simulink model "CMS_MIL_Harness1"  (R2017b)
settings: Solver=FixedStepDiscrete  StartTime=0.0  StopTime=23  FixedStep=0.01  RelTol=1e-3  EnableMultiTasking=on
undefined symbols (not defined in the file): sigbuilder_block
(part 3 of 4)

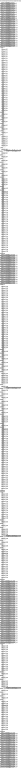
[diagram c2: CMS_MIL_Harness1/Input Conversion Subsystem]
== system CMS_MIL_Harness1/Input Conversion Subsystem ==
  note: This subsystem has been inserted by Simulink to adapt the output of the source blocks to the interface required by the harnessed component. Modifying the contents of this subsystem may result in compilation and simulation failure.
  Inport_1 : Inport
  Inport_2 : Inport  Port=2
  Inport_3 : Inport  Port=3
  Inport_4 : Inport  Port=4
  Inport_5 : Inport  Port=5
  Inport_6 : Inport  Port=6
  Inport_7 : Inport  Port=7
  Inport_8 : Inport  Port=8
  Inport_9 : Inport  Port=9
  Inport_10 : Inport  Port=10
  Inport_11 : Inport  Port=11
  Inport_12 : Inport  Port=12
  Inport_13 : Inport  Port=13
  Inport_14 : Inport  Port=14
  Inport_15 : Inport  Port=15
  Inport_16 : Inport  Port=16
  Inport_17 : Inport  Port=17
  Inport_18 : Inport  Port=18
  Inport_19 : Inport  Port=19
  Inport_20 : Inport  Port=20
  Inport_21 : Inport  Port=21
  Inport_22 : Inport  Port=22
  Inport_23 : Inport  Port=23
  Inport_24 : Inport  Port=24
  Inport_25 : Inport  Port=25
  Inport_26 : Inport  Port=26
  Inport_27 : Inport  Port=27
  Inport_28 : Inport  Port=28
  Inport_29 : Inport  Port=29
  Inport_30 : Inport  Port=30
  Inport_31 : Inport  Port=31
  Inport_32 : Inport  Port=32
  Inport_33 : Inport  Port=33
  Inport_34 : Inport  Port=34
  Inport_35 : Inport  Port=35
  Inport_36 : Inport  Port=36
  Inport_37 : Inport  Port=37
  Inport_38 : Inport  Port=38
  Inport_39 : Inport  Port=39
  Inport_40 : Inport  Port=40
  Inport_41 : Inport  Port=41
  Inport_42 : Inport  Port=42
  Inport_43 : Inport  Port=43
  Inport_44 : Inport  Port=44
  Inport_45 : Inport  Port=45
  Inport_46 : Inport  Port=46
  Inport_47 : Inport  Port=47
  Inport_48 : Inport  Port=48
  Inport_49 : Inport  Port=49
  Inport_50 : Inport  Port=50
  Inport_51 : Inport  Port=51
  Inport_52 : Inport  Port=52
  Inport_53 : Inport  Port=53
  Inport_54 : Inport  Port=54
  Inport_55 : Inport  Port=55
  Inport_56 : Inport  Port=56
  Inport_57 : Inport  Port=57
  Inport_58 : Inport  Port=58
  Inport_59 : Inport  Port=59
  Inport_60 : Inport  Port=60
  Inport_61 : Inport  Port=61
  Inport_62 : Inport  Port=62
  Inport_63 : Inport  Port=63
  Inport_64 : Inport  Port=64
  Inport_65 : Inport  Port=65
  Inport_66 : Inport  Port=66
  Inport_67 : Inport  Port=67
  Inport_68 : Inport  Port=68
  Inport_69 : Inport  Port=69
  Inport_70 : Inport  Port=70
  Inport_71 : Inport  Port=71
  Inport_72 : Inport  Port=72
  Inport_73 : Inport  Port=73
  Inport_74 : Inport  Port=74
  Inport_75 : Inport  Port=75
  Inport_76 : Inport  Port=76
  Inport_77 : Inport  Port=77
  Inport_78 : Inport  Port=78
  Inport_79 : Inport  Port=79
  Inport_80 : Inport  Port=80
  Inport_81 : Inport  Port=81
  Inport_82 : Inport  Port=82
  Inport_83 : Inport  Port=83
  Inport_84 : Inport  Port=84
  Inport_85 : Inport  Port=85
  Inport_86 : Inport  Port=86
  Inport_87 : Inport  Port=87
  Inport_88 : Inport  Port=88
  Inport_89 : Inport  Port=89
  Inport_90 : Inport  Port=90
  Inport_91 : Inport  Port=91
  Inport_92 : Inport  Port=92
  Inport_93 : Inport  Port=93
  Inport_94 : Inport  Port=94
  Inport_95 : Inport  Port=95
  Inport_96 : Inport  Port=96
  Inport_97 : Inport  Port=97
  Inport_98 : Inport  Port=98
  Inport_99 : Inport  Port=99
  Inport_100 : Inport  Port=100
  Inport_101 : Inport  Port=101
  Inport_102 : Inport  Port=102
  Inport_103 : Inport  Port=103
  Inport_104 : Inport  Port=104
  Inport_105 : Inport  Port=105
  Inport_106 : Inport  Port=106
  Inport_107 : Inport  Port=107
  Inport_108 : Inport  Port=108
  Inport_109 : Inport  Port=109
  Inport_110 : Inport  Port=110
  Inport_111 : Inport  Port=111
  Inport_112 : Inport  Port=112
  Inport_113 : Inport  Port=113
  Inport_114 : Inport  Port=114
  Inport_115 : Inport  Port=115
  Inport_116 : Inport  Port=116
  Inport_117 : Inport  Port=117
  Inport_118 : Inport  Port=118
  Inport_119 : Inport  Port=119
  Inport_120 : Inport  Port=120
  Inport_121 : Inport  Port=121
  Inport_122 : Inport  Port=122
  Inport_123 : Inport  Port=123
  Inport_124 : Inport  Port=124
  Inport_125 : Inport  Port=125
  Inport_126 : Inport  Port=126
  Inport_127 : Inport  Port=127
  Inport_128 : Inport  Port=128
  Inport_129 : Inport  Port=129
  Inport_130 : Inport  Port=130
  Inport_131 : Inport  Port=131
  Inport_132 : Inport  Port=132
  Inport_133 : Inport  Port=133
  Inport_134 : Inport  Port=134
  Inport_135 : Inport  Port=135
  Inport_136 : Inport  Port=136
  Inport_137 : Inport  Port=137
  Inport_138 : Inport  Port=138
  Inport_139 : Inport  Port=139
  Inport_140 : Inport  Port=140
  Inport_141 : Inport  Port=141
  Inport_142 : Inport  Port=142
  Inport_143 : Inport  Port=143
  Inport_144 : Inport  Port=144
  Inport_145 : Inport  Port=145
  Inport_146 : Inport  Port=146
  Inport_147 : Inport  Port=147
  Inport_148 : Inport  Port=148
  Inport_149 : Inport  Port=149
  Inport_150 : Inport  Port=150
  Inport_151 : Inport  Port=151
  Inport_152 : Inport  Port=152
  Inport_153 : Inport  Port=153
  Inport_154 : Inport  Port=154
  Inport_155 : Inport  Port=155
  Inport_156 : Inport  Port=156
  Inport_157 : Inport  Port=157
  Inport_158 : Inport  Port=158
  Inport_159 : Inport  Port=159
  Inport_160 : Inport  Port=160
  Inport_161 : Inport  Port=161
  Inport_162 : Inport  Port=162
  Inport_163 : Inport  Port=163
  Inport_164 : Inport  Port=164
  Inport_165 : Inport  Port=165
  Inport_166 : Inport  Port=166
  Inport_167 : Inport  Port=167
  Inport_168 : Inport  Port=168
  Inport_169 : Inport  Port=169
  Inport_170 : Inport  Port=170
  Inport_171 : Inport  Port=171
  Inport_172 : Inport  Port=172
  Inport_173 : Inport  Port=173
  Inport_174 : Inport  Port=174
  Inport_175 : Inport  Port=175
  Inport_176 : Inport  Port=176
  Inport_177 : Inport  Port=177
  Inport_178 : Inport  Port=178
  Inport_179 : Inport  Port=179
  Inport_180 : Inport  Port=180
  Inport_181 : Inport  Port=181
  Inport_182 : Inport  Port=182
  Inport_183 : Inport  Port=183
  Inport_184 : Inport  Port=184
  Inport_185 : Inport  Port=185
  Inport_186 : Inport  Port=186
  Inport_187 : Inport  Port=187
  Inport_188 : Inport  Port=188
  Inport_189 : Inport  Port=189
  Inport_190 : Inport  Port=190
  Inport_191 : Inport  Port=191
  Inport_192 : Inport  Port=192
  Inport_193 : Inport  Port=193
  Inport_194 : Inport  Port=194
  Inport_195 : Inport  Port=195
  Inport_196 : Inport  Port=196
  Inport_197 : Inport  Port=197
  Inport_198 : Inport  Port=198
  Inport_199 : Inport  Port=199
  Inport_200 : Inport  Port=200
  Inport_201 : Inport  Port=201
  Inport_202 : Inport  Port=202
  Inport_203 : Inport  Port=203
  Inport_204 : Inport  Port=204
  Inport_205 : Inport  Port=205
  Inport_206 : Inport  Port=206
  Inport_207 : Inport  Port=207
  Inport_208 : Inport  Port=208
  Inport_209 : Inport  Port=209
  Inport_210 : Inport  Port=210
  Inport_211 : Inport  Port=211
  Inport_212 : Inport  Port=212
  Inport_213 : Inport  Port=213
  Inport_214 : Inport  Port=214
  Inport_215 : Inport  Port=215
  Inport_216 : Inport  Port=216
  Inport_217 : Inport  Port=217
  Inport_218 : Inport  Port=218
  Inport_219 : Inport  Port=219
  Inport_220 : Inport  Port=220
  Inport_221 : Inport  Port=221
  Inport_222 : Inport  Port=222
  Inport_223 : Inport  Port=223
  Inport_224 : Inport  Port=224
  Inport_225 : Inport  Port=225
  Inport_226 : Inport  Port=226
  Inport_227 : Inport  Port=227
  Inport_228 : Inport  Port=228
  Inport_229 : Inport  Port=229
  Inport_230 : Inport  Port=230
  Inport_231 : Inport  Port=231
  Inport_232 : Inport  Port=232
  Inport_233 : Inport  Port=233
  Inport_234 : Inport  Port=234
  Inport_235 : Inport  Port=235
  Inport_236 : Inport  Port=236
  Inport_237 : Inport  Port=237
  Inport_238 : Inport  Port=238
  Inport_239 : Inport  Port=239
  Inport_240 : Inport  Port=240
  Inport_241 : Inport  Port=241
  Inport_242 : Inport  Port=242
  Inport_243 : Inport  Port=243
  Inport_244 : Inport  Port=244
  Inport_245 : Inport  Port=245
  Inport_246 : Inport  Port=246
  Inport_247 : Inport  Port=247
  Inport_248 : Inport  Port=248
  Inport_249 : Inport  Port=249
  Inport_250 : Inport  Port=250
  Inport_251 : Inport  Port=251
  Inport_252 : Inport  Port=252
  Inport_253 : Inport  Port=253
  Inport_254 : Inport  Port=254
  Inport_255 : Inport  Port=255
  Inport_256 : Inport  Port=256
  Inport_257 : Inport  Port=257
  Inport_258 : Inport  Port=258
  Inport_259 : Inport  Port=259
  Inport_260 : Inport  Port=260
  Inport_261 : Inport  Port=261
  Inport_262 : Inport  Port=262
  Inport_263 : Inport  Port=263
  Inport_264 : Inport  Port=264
  Inport_265 : Inport  Port=265
  Inport_266 : Inport  Port=266
  Inport_267 : Inport  Port=267
  Inport_268 : Inport  Port=268
  Inport_269 : Inport  Port=269
  Inport_270 : Inport  Port=270
  Inport_271 : Inport  Port=271
  Inport_272 : Inport  Port=272
  Inport_273 : Inport  Port=273
  Inport_274 : Inport  Port=274
  Inport_275 : Inport  Port=275
  Inport_276 : Inport  Port=276
  Inport_277 : Inport  Port=277
  Inport_278 : Inport  Port=278
  Inport_279 : Inport  Port=279
  Inport_280 : Inport  Port=280
  Inport_281 : Inport  Port=281
  Inport_282 : Inport  Port=282
  Inport_283 : Inport  Port=283
  Inport_284 : Inport  Port=284
  Inport_285 : Inport  Port=285
  Inport_286 : Inport  Port=286
  Inport_287 : Inport  Port=287
  Inport_288 : Inport  Port=288
  Inport_289 : Inport  Port=289
  Inport_290 : Inport  Port=290
  Inport_291 : Inport  Port=291
  Inport_292 : Inport  Port=292
  Inport_293 : Inport  Port=293
  Inport_294 : Inport  Port=294
  Inport_295 : Inport  Port=295
  Inport_296 : Inport  Port=296
  Inport_297 : Inport  Port=297
  Inport_298 : Inport  Port=298
  Inport_299 : Inport  Port=299
  Inport_300 : Inport  Port=300
  Inport_301 : Inport  Port=301
  Inport_302 : Inport  Port=302
  Inport_303 : Inport  Port=303
  Inport_304 : Inport  Port=304
  Inport_305 : Inport  Port=305
  Inport_306 : Inport  Port=306
  Inport_307 : Inport  Port=307
  Inport_308 : Inport  Port=308
  Inport_309 : Inport  Port=309
  Inport_310 : Inport  Port=310
  Inport_311 : Inport  Port=311
  Inport_312 : Inport  Port=312
  Inport_313 : Inport  Port=313
  Inport_314 : Inport  Port=314
  Inport_315 : Inport  Port=315
  Inport_316 : Inport  Port=316
  Inport_317 : Inport  Port=317
  Inport_318 : Inport  Port=318
  Inport_319 : Inport  Port=319
  Inport_320 : Inport  Port=320
  Inport_321 : Inport  Port=321
  Inport_322 : Inport  Port=322
  Inport_323 : Inport  Port=323
  Inport_324 : Inport  Port=324
  Inport_325 : Inport  Port=325
  Inport_326 : Inport  Port=326
  Inport_327 : Inport  Port=327
  Inport_328 : Inport  Port=328
  Inport_329 : Inport  Port=329
  Inport_330 : Inport  Port=330
  Inport_331 : Inport  Port=331
  Inport_332 : Inport  Port=332
  Inport_333 : Inport  Port=333
  Inport_334 : Inport  Port=334
  Inport_335 : Inport  Port=335
  Inport_336 : Inport  Port=336
  Inport_337 : Inport  Port=337
  Inport_338 : Inport  Port=338
  Inport_339 : Inport  Port=339
  Inport_340 : Inport  Port=340
  Inport_341 : Inport  Port=341
  Inport_342 : Inport  Port=342
  Inport_343 : Inport  Port=343
  Inport_344 : Inport  Port=344
  Inport_345 : Inport  Port=345
  Inport_346 : Inport  Port=346
  Inport_347 : Inport  Port=347
  Inport_348 : Inport  Port=348
  Inport_349 : Inport  Port=349
  Inport_350 : Inport  Port=350
  Inport_351 : Inport  Port=351
  Inport_352 : Inport  Port=352
  Inport_353 : Inport  Port=353
  Inport_354 : Inport  Port=354
  Inport_355 : Inport  Port=355
  Inport_356 : Inport  Port=356
  Inport_357 : Inport  Port=357
  Inport_358 : Inport  Port=358
  Inport_359 : Inport  Port=359
  Inport_360 : Inport  Port=360
  Inport_361 : Inport  Port=361
  Inport_362 : Inport  Port=362
  Inport_363 : Inport  Port=363
  Inport_364 : Inport  Port=364
  Inport_365 : Inport  Port=365
  Inport_366 : Inport  Port=366
  Inport_367 : Inport  Port=367
  Inport_368 : Inport  Port=368
  Inport_369 : Inport  Port=369
  Inport_370 : Inport  Port=370
  Inport_371 : Inport  Port=371
  Inport_372 : Inport  Port=372
  Inport_373 : Inport  Port=373
  Inport_374 : Inport  Port=374
  Inport_375 : Inport  Port=375
  Inport_376 : Inport  Port=376
  Inport_377 : Inport  Port=377
  Inport_378 : Inport  Port=378
  Inport_379 : Inport  Port=379
  Inport_380 : Inport  Port=380
  Inport_381 : Inport  Port=381
  Inport_382 : Inport  Port=382
  Inport_383 : Inport  Port=383
  Inport_384 : Inport  Port=384
  Inport_385 : Inport  Port=385
  Inport_386 : Inport  Port=386
  Inport_387 : Inport  Port=387
  Inport_388 : Inport  Port=388
  Inport_389 : Inport  Port=389
  Inport_390 : Inport  Port=390
  Inport_391 : Inport  Port=391
  Inport_392 : Inport  Port=392
  Inport_393 : Inport  Port=393
  Inport_394 : Inport  Port=394
  Inport_395 : Inport  Port=395
  Inport_396 : Inport  Port=396
  Inport_397 : Inport  Port=397
  Inport_398 : Inport  Port=398
  Inport_399 : Inport  Port=399
  Inport_400 : Inport  Port=400
  Inport_401 : Inport  Port=401
  Inport_402 : Inport  Port=402
  Inport_403 : Inport  Port=403
  Inport_404 : Inport  Port=404
  Inport_405 : Inport  Port=405
  Inport_406 : Inport  Port=406
  Inport_407 : Inport  Port=407
  Inport_408 : Inport  Port=408
  Inport_409 : Inport  Port=409
  Inport_410 : Inport  Port=410
  Inport_411 : Inport  Port=411
  Inport_412 : Inport  Port=412
  Inport_413 : Inport  Port=413
  Concat_1 : Concatenate  NumInputs=112
  Concat_2 : Concatenate  NumInputs=112
  Concat_3 : Concatenate  NumInputs=48
  Concat_4 : Concatenate  NumInputs=48
  Data_Conversion_{1,16,20,31,34..36,51..52,54,58..61,73,78..79,83..85,99..101} (23 alike) : DataTypeConversion  OutDataTypeStr=uint8
  Data_Conversion_{10..11,30,43,71..72,86} (7 alike) : DataTypeConversion  OutDataTypeStr=uint16
  Data_Conversion_{2..5,7,9,12,15,17,19,24..25,27,32..33,38,53,56,62..64,67..68,80,87..88,91..98} (34 alike) : DataTypeConversion  OutDataTypeStr=boolean
  Data_Conversion_{6,8,13..14,18,21..23,28..29,37,39..40,42,45,47..50,55,57,65..66,69..70,74..77,81,89..90} (32 alike) : DataTypeConversion  OutDataTypeStr=single
  Data_Conversion_26 : Reshape  OutputDimensionality=Customize  OutputDimensions=[112]
  Data_Conversion_41 : DataTypeConversion  OutDataTypeStr=fixdt('ufix16_Sp1')
  Data_Conversion_44 : Reshape  OutputDimensionality=Customize  OutputDimensions=[112]
  Data_Conversion_46 : Reshape  OutputDimensionality=Customize  OutputDimensions=[48]
  Data_Conversion_82 : Reshape  OutputDimensionality=Customize  OutputDimensions=[48]
  RateTs_{1..97} (97 alike) : RateTransition  OutPortSampleTime=0.01
  SigSpec_{1,16,20,33..35,48..49,51,70,75,95..97} (14 alike) : SignalSpecification  OutDataTypeStr=uint8  Unit=enum  Dimensions=[1]  SampleTime=0.01
  SigSpec_10 : SignalSpecification  OutDataTypeStr=uint16  Unit=mV  Dimensions=[1]  SampleTime=0.01
  SigSpec_11 : SignalSpecification  OutDataTypeStr=uint16  Unit=mV  Dimensions=[1]  SampleTime=0.01
  SigSpec_{12,15,17,19,24,26,31..32,37,50,60..61,64..65,77,83..84,87..93} (24 alike) : SignalSpecification  OutDataTypeStr=boolean  Unit=flag  Dimensions=[1]  SampleTime=0.01
  SigSpec_{6,13,52,54,63,85} (6 alike) : SignalSpecification  OutDataTypeStr=single  Unit=V  Dimensions=[1]  SampleTime=0.01
  SigSpec_{8,14,23,41,62,86} (6 alike) : SignalSpecification  OutDataTypeStr=single  Unit=A  Dimensions=[1]  SampleTime=0.01
  SigSpec_18 : SignalSpecification  OutDataTypeStr=single  Unit=pct  Dimensions=[1]  SampleTime=0.01
  SigSpec_{2..5,7,9,53,59,94} (9 alike) : SignalSpecification  OutDataTypeStr=boolean  Unit=flg  Dimensions=[1]  SampleTime=0.01
  SigSpec_21 : SignalSpecification  OutDataTypeStr=single  Unit=pct  Dimensions=[1]  SampleTime=0.01
  SigSpec_22 : SignalSpecification  OutDataTypeStr=single  Unit=pct  Dimensions=[1]  SampleTime=0.01
  SigSpec_25 : SignalSpecification  OutDataTypeStr=boolean  Unit=flag  Dimensions=[112]  SampleTime=0.01
  SigSpec_{27..28,71..72} (4 alike) : SignalSpecification  OutDataTypeStr=single  Unit=kW  Dimensions=[1]  SampleTime=0.01
  SigSpec_29 : SignalSpecification  OutDataTypeStr=uint16  Unit=kohm  Dimensions=[1]  SampleTime=0.01
  SigSpec_{30,55..58,76,79..81} (9 alike) : SignalSpecification  OutDataTypeStr=uint8  Unit=numb  Dimensions=[1]  SampleTime=0.01
  SigSpec_{36,38..39,44..45,66..67,73..74} (9 alike) : SignalSpecification  OutDataTypeStr=single  Unit=C  Dimensions=[1]  SampleTime=0.01
  SigSpec_40 : SignalSpecification  OutDataTypeStr=fixdt('ufix16_Sp1')  Unit=V  Dimensions=[1]  SampleTime=0.01
  SigSpec_42 : SignalSpecification  OutDataTypeStr=uint16  Unit=mV  Dimensions=[112]  SampleTime=0.01
  SigSpec_43 : SignalSpecification  OutDataTypeStr=single  Unit=C  Dimensions=[48]  SampleTime=0.01
  SigSpec_46 : SignalSpecification  OutDataTypeStr=single  Unit=W  Dimensions=[1]  SampleTime=0.01
  SigSpec_47 : SignalSpecification  OutDataTypeStr=single  Unit=W  Dimensions=[1]  SampleTime=0.01
  SigSpec_68 : SignalSpecification  OutDataTypeStr=uint16  Unit=min  Dimensions=[1]  SampleTime=0.01
  SigSpec_69 : SignalSpecification  OutDataTypeStr=uint16  Unit=min  Dimensions=[1]  SampleTime=0.01
  SigSpec_78 : SignalSpecification  OutDataTypeStr=single  Unit=C  Dimensions=[48]  SampleTime=0.01
  SigSpec_82 : SignalSpecification  OutDataTypeStr=uint16  Unit=kWh  Dimensions=[1]  SampleTime=0.01
  Outport_1 : Outport
  Outport_2 : Outport  Port=2
  Outport_3 : Outport  Port=3
  Outport_4 : Outport  Port=4
  Outport_5 : Outport  Port=5
  Outport_6 : Outport  Port=6
  Outport_7 : Outport  Port=7
  Outport_8 : Outport  Port=8
  Outport_9 : Outport  Port=9
  Outport_10 : Outport  Port=10
  Outport_11 : Outport  Port=11
  Outport_12 : Outport  Port=12
  Outport_13 : Outport  Port=13
  Outport_14 : Outport  Port=14
  Outport_15 : Outport  Port=15
  Outport_16 : Outport  Port=16
  Outport_17 : Outport  Port=17
  Outport_18 : Outport  Port=18
  Outport_19 : Outport  Port=19
  Outport_20 : Outport  Port=20
  Outport_21 : Outport  Port=21
  Outport_22 : Outport  Port=22
  Outport_23 : Outport  Port=23
  Outport_24 : Outport  Port=24
  Outport_25 : Outport  Port=25
  Outport_26 : Outport  Port=26
  Outport_27 : Outport  Port=27
  Outport_28 : Outport  Port=28
  Outport_29 : Outport  Port=29
  Outport_30 : Outport  Port=30
  Outport_31 : Outport  Port=31
  Outport_32 : Outport  Port=32
  Outport_33 : Outport  Port=33
  Outport_34 : Outport  Port=34
  Outport_35 : Outport  Port=35
  Outport_36 : Outport  Port=36
  Outport_37 : Outport  Port=37
  Outport_38 : Outport  Port=38
  Outport_39 : Outport  Port=39
  Outport_40 : Outport  Port=40
  Outport_41 : Outport  Port=41
  Outport_42 : Outport  Port=42
  Outport_43 : Outport  Port=43
  Outport_44 : Outport  Port=44
  Outport_45 : Outport  Port=45
  Outport_46 : Outport  Port=46
  Outport_47 : Outport  Port=47
  Outport_48 : Outport  Port=48
  Outport_49 : Outport  Port=49
  Outport_50 : Outport  Port=50
  Outport_51 : Outport  Port=51
  Outport_52 : Outport  Port=52
  Outport_53 : Outport  Port=53
  Outport_54 : Outport  Port=54
  Outport_55 : Outport  Port=55
  Outport_56 : Outport  Port=56
  Outport_57 : Outport  Port=57
  Outport_58 : Outport  Port=58
  Outport_59 : Outport  Port=59
  Outport_60 : Outport  Port=60
  Outport_61 : Outport  Port=61
  Outport_62 : Outport  Port=62
  Outport_63 : Outport  Port=63
  Outport_64 : Outport  Port=64
  Outport_65 : Outport  Port=65
  Outport_66 : Outport  Port=66
  Outport_67 : Outport  Port=67
  Outport_68 : Outport  Port=68
  Outport_69 : Outport  Port=69
  Outport_70 : Outport  Port=70
  Outport_71 : Outport  Port=71
  Outport_72 : Outport  Port=72
  Outport_73 : Outport  Port=73
  Outport_74 : Outport  Port=74
  Outport_75 : Outport  Port=75
  Outport_76 : Outport  Port=76
  Outport_77 : Outport  Port=77
  Outport_78 : Outport  Port=78
  Outport_79 : Outport  Port=79
  Outport_80 : Outport  Port=80
  Outport_81 : Outport  Port=81
  Outport_82 : Outport  Port=82
  Outport_83 : Outport  Port=83
  Outport_84 : Outport  Port=84
  Outport_85 : Outport  Port=85
  Outport_86 : Outport  Port=86
  Outport_87 : Outport  Port=87
  Outport_88 : Outport  Port=88
  Outport_89 : Outport  Port=89
  Outport_90 : Outport  Port=90
  Outport_91 : Outport  Port=91
  Outport_92 : Outport  Port=92
  Outport_93 : Outport  Port=93
  Outport_94 : Outport  Port=94
  Outport_95 : Outport  Port=95
  Outport_96 : Outport  Port=96
  Outport_97 : Outport  Port=97
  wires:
  SigSpec_1/1 -> Outport_1/1
  RateTs_1/1 -> SigSpec_1/1
  Data_Conversion_1/1 -> RateTs_1/1
  Inport_1/1 -> Data_Conversion_1/1
  SigSpec_2/1 -> Outport_2/1
  RateTs_2/1 -> SigSpec_2/1
  Data_Conversion_2/1 -> RateTs_2/1
  Inport_2/1 -> Data_Conversion_2/1
  SigSpec_3/1 -> Outport_3/1
  RateTs_3/1 -> SigSpec_3/1
  Data_Conversion_3/1 -> RateTs_3/1
  Inport_3/1 -> Data_Conversion_3/1
  SigSpec_4/1 -> Outport_4/1
  RateTs_4/1 -> SigSpec_4/1
  Data_Conversion_4/1 -> RateTs_4/1
  Inport_4/1 -> Data_Conversion_4/1
  SigSpec_5/1 -> Outport_5/1
  RateTs_5/1 -> SigSpec_5/1
  Data_Conversion_5/1 -> RateTs_5/1
  Inport_5/1 -> Data_Conversion_5/1
  SigSpec_6/1 -> Outport_6/1
  RateTs_6/1 -> SigSpec_6/1
  Data_Conversion_6/1 -> RateTs_6/1
  Inport_6/1 -> Data_Conversion_6/1
  SigSpec_7/1 -> Outport_7/1
  RateTs_7/1 -> SigSpec_7/1
  Data_Conversion_7/1 -> RateTs_7/1
  Inport_7/1 -> Data_Conversion_7/1
  SigSpec_8/1 -> Outport_8/1
  RateTs_8/1 -> SigSpec_8/1
  Data_Conversion_8/1 -> RateTs_8/1
  Inport_8/1 -> Data_Conversion_8/1
  SigSpec_9/1 -> Outport_9/1
  RateTs_9/1 -> SigSpec_9/1
  Data_Conversion_9/1 -> RateTs_9/1
  Inport_9/1 -> Data_Conversion_9/1
  SigSpec_10/1 -> Outport_10/1
  RateTs_10/1 -> SigSpec_10/1
  Data_Conversion_10/1 -> RateTs_10/1
  Inport_10/1 -> Data_Conversion_10/1
  SigSpec_11/1 -> Outport_11/1
  RateTs_11/1 -> SigSpec_11/1
  Data_Conversion_11/1 -> RateTs_11/1
  Inport_11/1 -> Data_Conversion_11/1
  SigSpec_12/1 -> Outport_12/1
  RateTs_12/1 -> SigSpec_12/1
  Data_Conversion_12/1 -> RateTs_12/1
  Inport_12/1 -> Data_Conversion_12/1
  SigSpec_13/1 -> Outport_13/1
  RateTs_13/1 -> SigSpec_13/1
  Data_Conversion_13/1 -> RateTs_13/1
  Inport_13/1 -> Data_Conversion_13/1
  SigSpec_14/1 -> Outport_14/1
  RateTs_14/1 -> SigSpec_14/1
  Data_Conversion_14/1 -> RateTs_14/1
  Inport_14/1 -> Data_Conversion_14/1
  SigSpec_15/1 -> Outport_15/1
  RateTs_15/1 -> SigSpec_15/1
  Data_Conversion_15/1 -> RateTs_15/1
  Inport_15/1 -> Data_Conversion_15/1
  SigSpec_16/1 -> Outport_16/1
  RateTs_16/1 -> SigSpec_16/1
  Data_Conversion_16/1 -> RateTs_16/1
  Inport_16/1 -> Data_Conversion_16/1
  SigSpec_17/1 -> Outport_17/1
  RateTs_17/1 -> SigSpec_17/1
  Data_Conversion_17/1 -> RateTs_17/1
  Inport_17/1 -> Data_Conversion_17/1
  SigSpec_18/1 -> Outport_18/1
  RateTs_18/1 -> SigSpec_18/1
  Data_Conversion_18/1 -> RateTs_18/1
  Inport_18/1 -> Data_Conversion_18/1
  SigSpec_19/1 -> Outport_19/1
  RateTs_19/1 -> SigSpec_19/1
  Data_Conversion_19/1 -> RateTs_19/1
  Inport_19/1 -> Data_Conversion_19/1
  SigSpec_20/1 -> Outport_20/1
  RateTs_20/1 -> SigSpec_20/1
  Data_Conversion_20/1 -> RateTs_20/1
  Inport_20/1 -> Data_Conversion_20/1
  SigSpec_21/1 -> Outport_21/1
  RateTs_21/1 -> SigSpec_21/1
  Data_Conversion_21/1 -> RateTs_21/1
  Inport_21/1 -> Data_Conversion_21/1
  SigSpec_22/1 -> Outport_22/1
  RateTs_22/1 -> SigSpec_22/1
  Data_Conversion_22/1 -> RateTs_22/1
  Inport_22/1 -> Data_Conversion_22/1
  SigSpec_23/1 -> Outport_23/1
  RateTs_23/1 -> SigSpec_23/1
  Data_Conversion_23/1 -> RateTs_23/1
  Inport_23/1 -> Data_Conversion_23/1
  SigSpec_24/1 -> Outport_24/1
  RateTs_24/1 -> SigSpec_24/1
  Data_Conversion_24/1 -> RateTs_24/1
  Inport_24/1 -> Data_Conversion_24/1
  SigSpec_25/1 -> Outport_25/1
  RateTs_25/1 -> SigSpec_25/1
  Data_Conversion_25/1 -> RateTs_25/1
  Data_Conversion_26/1 -> Data_Conversion_25/1
  Concat_1/1 -> Data_Conversion_26/1
  Inport_25/1 -> Concat_1/1
  Inport_26/1 -> Concat_1/2
  Inport_27/1 -> Concat_1/3
  Inport_28/1 -> Concat_1/4
  Inport_29/1 -> Concat_1/5
  Inport_30/1 -> Concat_1/6
  Inport_31/1 -> Concat_1/7
  Inport_32/1 -> Concat_1/8
  Inport_33/1 -> Concat_1/9
  Inport_34/1 -> Concat_1/10
  Inport_35/1 -> Concat_1/11
  Inport_36/1 -> Concat_1/12
  Inport_37/1 -> Concat_1/13
  Inport_38/1 -> Concat_1/14
  Inport_39/1 -> Concat_1/15
  Inport_40/1 -> Concat_1/16
  Inport_41/1 -> Concat_1/17
  Inport_42/1 -> Concat_1/18
  Inport_43/1 -> Concat_1/19
  Inport_44/1 -> Concat_1/20
  Inport_45/1 -> Concat_1/21
  Inport_46/1 -> Concat_1/22
  Inport_47/1 -> Concat_1/23
  Inport_48/1 -> Concat_1/24
  Inport_49/1 -> Concat_1/25
  Inport_50/1 -> Concat_1/26
  Inport_51/1 -> Concat_1/27
  Inport_52/1 -> Concat_1/28
  Inport_53/1 -> Concat_1/29
  Inport_54/1 -> Concat_1/30
  Inport_55/1 -> Concat_1/31
  Inport_56/1 -> Concat_1/32
  Inport_57/1 -> Concat_1/33
  Inport_58/1 -> Concat_1/34
  Inport_59/1 -> Concat_1/35
  Inport_60/1 -> Concat_1/36
  Inport_61/1 -> Concat_1/37
  Inport_62/1 -> Concat_1/38
  Inport_63/1 -> Concat_1/39
  Inport_64/1 -> Concat_1/40
  Inport_65/1 -> Concat_1/41
  Inport_66/1 -> Concat_1/42
  Inport_67/1 -> Concat_1/43
  Inport_68/1 -> Concat_1/44
  Inport_69/1 -> Concat_1/45
  Inport_70/1 -> Concat_1/46
  Inport_71/1 -> Concat_1/47
  Inport_72/1 -> Concat_1/48
  Inport_73/1 -> Concat_1/49
  Inport_74/1 -> Concat_1/50
  Inport_75/1 -> Concat_1/51
  Inport_76/1 -> Concat_1/52
  Inport_77/1 -> Concat_1/53
  Inport_78/1 -> Concat_1/54
  Inport_79/1 -> Concat_1/55
  Inport_80/1 -> Concat_1/56
  Inport_81/1 -> Concat_1/57
  Inport_82/1 -> Concat_1/58
  Inport_83/1 -> Concat_1/59
  Inport_84/1 -> Concat_1/60
  Inport_85/1 -> Concat_1/61
  Inport_86/1 -> Concat_1/62
  Inport_87/1 -> Concat_1/63
  Inport_88/1 -> Concat_1/64
  Inport_89/1 -> Concat_1/65
  Inport_90/1 -> Concat_1/66
  Inport_91/1 -> Concat_1/67
  Inport_92/1 -> Concat_1/68
  Inport_93/1 -> Concat_1/69
  Inport_94/1 -> Concat_1/70
  Inport_95/1 -> Concat_1/71
  Inport_96/1 -> Concat_1/72
  Inport_97/1 -> Concat_1/73
  Inport_98/1 -> Concat_1/74
  Inport_99/1 -> Concat_1/75
  Inport_100/1 -> Concat_1/76
  Inport_101/1 -> Concat_1/77
  Inport_102/1 -> Concat_1/78
  Inport_103/1 -> Concat_1/79
  Inport_104/1 -> Concat_1/80
  Inport_105/1 -> Concat_1/81
  Inport_106/1 -> Concat_1/82
  Inport_107/1 -> Concat_1/83
  Inport_108/1 -> Concat_1/84
  Inport_109/1 -> Concat_1/85
  Inport_110/1 -> Concat_1/86
  Inport_111/1 -> Concat_1/87
  Inport_112/1 -> Concat_1/88
  Inport_113/1 -> Concat_1/89
  Inport_114/1 -> Concat_1/90
  Inport_115/1 -> Concat_1/91
  Inport_116/1 -> Concat_1/92
  Inport_117/1 -> Concat_1/93
  Inport_118/1 -> Concat_1/94
  Inport_119/1 -> Concat_1/95
  Inport_120/1 -> Concat_1/96
  Inport_121/1 -> Concat_1/97
  Inport_122/1 -> Concat_1/98
  Inport_123/1 -> Concat_1/99
  Inport_124/1 -> Concat_1/100
  Inport_125/1 -> Concat_1/101
  Inport_126/1 -> Concat_1/102
  Inport_127/1 -> Concat_1/103
  Inport_128/1 -> Concat_1/104
  Inport_129/1 -> Concat_1/105
  Inport_130/1 -> Concat_1/106
  Inport_131/1 -> Concat_1/107
  Inport_132/1 -> Concat_1/108
  Inport_133/1 -> Concat_1/109
  Inport_134/1 -> Concat_1/110
  Inport_135/1 -> Concat_1/111
  Inport_136/1 -> Concat_1/112
  SigSpec_26/1 -> Outport_26/1
  RateTs_26/1 -> SigSpec_26/1
  Data_Conversion_27/1 -> RateTs_26/1
  Inport_137/1 -> Data_Conversion_27/1
  SigSpec_27/1 -> Outport_27/1
  RateTs_27/1 -> SigSpec_27/1
  Data_Conversion_28/1 -> RateTs_27/1
  Inport_138/1 -> Data_Conversion_28/1
  SigSpec_28/1 -> Outport_28/1
  RateTs_28/1 -> SigSpec_28/1
  Data_Conversion_29/1 -> RateTs_28/1
  Inport_139/1 -> Data_Conversion_29/1
  SigSpec_29/1 -> Outport_29/1
  RateTs_29/1 -> SigSpec_29/1
  Data_Conversion_30/1 -> RateTs_29/1
  Inport_140/1 -> Data_Conversion_30/1
  SigSpec_30/1 -> Outport_30/1
  RateTs_30/1 -> SigSpec_30/1
  Data_Conversion_31/1 -> RateTs_30/1
  Inport_141/1 -> Data_Conversion_31/1
  SigSpec_31/1 -> Outport_31/1
  RateTs_31/1 -> SigSpec_31/1
  Data_Conversion_32/1 -> RateTs_31/1
  Inport_142/1 -> Data_Conversion_32/1
  SigSpec_32/1 -> Outport_32/1
  RateTs_32/1 -> SigSpec_32/1
  Data_Conversion_33/1 -> RateTs_32/1
  Inport_143/1 -> Data_Conversion_33/1
  SigSpec_33/1 -> Outport_33/1
  RateTs_33/1 -> SigSpec_33/1
  Data_Conversion_34/1 -> RateTs_33/1
  Inport_144/1 -> Data_Conversion_34/1
  SigSpec_34/1 -> Outport_34/1
  RateTs_34/1 -> SigSpec_34/1
  Data_Conversion_35/1 -> RateTs_34/1
  Inport_145/1 -> Data_Conversion_35/1
  SigSpec_35/1 -> Outport_35/1
  RateTs_35/1 -> SigSpec_35/1
  Data_Conversion_36/1 -> RateTs_35/1
  Inport_146/1 -> Data_Conversion_36/1
  SigSpec_36/1 -> Outport_36/1
  RateTs_36/1 -> SigSpec_36/1
  Data_Conversion_37/1 -> RateTs_36/1
  Inport_147/1 -> Data_Conversion_37/1
  SigSpec_37/1 -> Outport_37/1
  RateTs_37/1 -> SigSpec_37/1
  Data_Conversion_38/1 -> RateTs_37/1
  Inport_148/1 -> Data_Conversion_38/1
  SigSpec_38/1 -> Outport_38/1
  RateTs_38/1 -> SigSpec_38/1
  Data_Conversion_39/1 -> RateTs_38/1
  Inport_149/1 -> Data_Conversion_39/1
  SigSpec_39/1 -> Outport_39/1
  RateTs_39/1 -> SigSpec_39/1
  Data_Conversion_40/1 -> RateTs_39/1
  Inport_150/1 -> Data_Conversion_40/1
  SigSpec_40/1 -> Outport_40/1
  RateTs_40/1 -> SigSpec_40/1
  Data_Conversion_41/1 -> RateTs_40/1
  Inport_151/1 -> Data_Conversion_41/1
  SigSpec_41/1 -> Outport_41/1
  RateTs_41/1 -> SigSpec_41/1
  Data_Conversion_42/1 -> RateTs_41/1
  Inport_152/1 -> Data_Conversion_42/1
  SigSpec_42/1 -> Outport_42/1
  RateTs_42/1 -> SigSpec_42/1
  Data_Conversion_43/1 -> RateTs_42/1
  Data_Conversion_44/1 -> Data_Conversion_43/1
  Concat_2/1 -> Data_Conversion_44/1
  Inport_153/1 -> Concat_2/1
  Inport_154/1 -> Concat_2/2
  Inport_155/1 -> Concat_2/3
  Inport_156/1 -> Concat_2/4
  Inport_157/1 -> Concat_2/5
  Inport_158/1 -> Concat_2/6
  Inport_159/1 -> Concat_2/7
  Inport_160/1 -> Concat_2/8
  Inport_161/1 -> Concat_2/9
  Inport_162/1 -> Concat_2/10
  Inport_163/1 -> Concat_2/11
  Inport_164/1 -> Concat_2/12
  Inport_165/1 -> Concat_2/13
  Inport_166/1 -> Concat_2/14
  Inport_167/1 -> Concat_2/15
  Inport_168/1 -> Concat_2/16
  Inport_169/1 -> Concat_2/17
  Inport_170/1 -> Concat_2/18
  Inport_171/1 -> Concat_2/19
  Inport_172/1 -> Concat_2/20
  Inport_173/1 -> Concat_2/21
  Inport_174/1 -> Concat_2/22
  Inport_175/1 -> Concat_2/23
  Inport_176/1 -> Concat_2/24
  Inport_177/1 -> Concat_2/25
  Inport_178/1 -> Concat_2/26
  Inport_179/1 -> Concat_2/27
  Inport_180/1 -> Concat_2/28
  Inport_181/1 -> Concat_2/29
  Inport_182/1 -> Concat_2/30
  Inport_183/1 -> Concat_2/31
  Inport_184/1 -> Concat_2/32
  Inport_185/1 -> Concat_2/33
  Inport_186/1 -> Concat_2/34
  Inport_187/1 -> Concat_2/35
  Inport_188/1 -> Concat_2/36
  Inport_189/1 -> Concat_2/37
  Inport_190/1 -> Concat_2/38
  Inport_191/1 -> Concat_2/39
  Inport_192/1 -> Concat_2/40
  Inport_193/1 -> Concat_2/41
  Inport_194/1 -> Concat_2/42
  Inport_195/1 -> Concat_2/43
  Inport_196/1 -> Concat_2/44
  Inport_197/1 -> Concat_2/45
  Inport_198/1 -> Concat_2/46
  Inport_199/1 -> Concat_2/47
  Inport_200/1 -> Concat_2/48
  Inport_201/1 -> Concat_2/49
  Inport_202/1 -> Concat_2/50
  Inport_203/1 -> Concat_2/51
  Inport_204/1 -> Concat_2/52
  Inport_205/1 -> Concat_2/53
  Inport_206/1 -> Concat_2/54
  Inport_207/1 -> Concat_2/55
  Inport_208/1 -> Concat_2/56
  Inport_209/1 -> Concat_2/57
  Inport_210/1 -> Concat_2/58
  Inport_211/1 -> Concat_2/59
  Inport_212/1 -> Concat_2/60
  Inport_213/1 -> Concat_2/61
  Inport_214/1 -> Concat_2/62
  Inport_215/1 -> Concat_2/63
  Inport_216/1 -> Concat_2/64
  Inport_217/1 -> Concat_2/65
  Inport_218/1 -> Concat_2/66
  Inport_219/1 -> Concat_2/67
  Inport_220/1 -> Concat_2/68
  Inport_221/1 -> Concat_2/69
  Inport_222/1 -> Concat_2/70
  Inport_223/1 -> Concat_2/71
  Inport_224/1 -> Concat_2/72
  Inport_225/1 -> Concat_2/73
  Inport_226/1 -> Concat_2/74
  Inport_227/1 -> Concat_2/75
  Inport_228/1 -> Concat_2/76
  Inport_229/1 -> Concat_2/77
  Inport_230/1 -> Concat_2/78
  Inport_231/1 -> Concat_2/79
  Inport_232/1 -> Concat_2/80
  Inport_233/1 -> Concat_2/81
  Inport_234/1 -> Concat_2/82
  Inport_235/1 -> Concat_2/83
  Inport_236/1 -> Concat_2/84
  Inport_237/1 -> Concat_2/85
  Inport_238/1 -> Concat_2/86
  Inport_239/1 -> Concat_2/87
  Inport_240/1 -> Concat_2/88
  Inport_241/1 -> Concat_2/89
  Inport_242/1 -> Concat_2/90
  Inport_243/1 -> Concat_2/91
  Inport_244/1 -> Concat_2/92
  Inport_245/1 -> Concat_2/93
  Inport_246/1 -> Concat_2/94
  Inport_247/1 -> Concat_2/95
  Inport_248/1 -> Concat_2/96
  Inport_249/1 -> Concat_2/97
  Inport_250/1 -> Concat_2/98
  Inport_251/1 -> Concat_2/99
  Inport_252/1 -> Concat_2/100
  Inport_253/1 -> Concat_2/101
  Inport_254/1 -> Concat_2/102
  Inport_255/1 -> Concat_2/103
  Inport_256/1 -> Concat_2/104
  Inport_257/1 -> Concat_2/105
  Inport_258/1 -> Concat_2/106
  Inport_259/1 -> Concat_2/107
  Inport_260/1 -> Concat_2/108
  Inport_261/1 -> Concat_2/109
  Inport_262/1 -> Concat_2/110
  Inport_263/1 -> Concat_2/111
  Inport_264/1 -> Concat_2/112
  SigSpec_43/1 -> Outport_43/1
  RateTs_43/1 -> SigSpec_43/1
  Data_Conversion_45/1 -> RateTs_43/1
  Data_Conversion_46/1 -> Data_Conversion_45/1
  Concat_3/1 -> Data_Conversion_46/1
  Inport_265/1 -> Concat_3/1
  Inport_266/1 -> Concat_3/2
  Inport_267/1 -> Concat_3/3
  Inport_268/1 -> Concat_3/4
  Inport_269/1 -> Concat_3/5
  Inport_270/1 -> Concat_3/6
  Inport_271/1 -> Concat_3/7
  Inport_272/1 -> Concat_3/8
  Inport_273/1 -> Concat_3/9
  Inport_274/1 -> Concat_3/10
  Inport_275/1 -> Concat_3/11
  Inport_276/1 -> Concat_3/12
  Inport_277/1 -> Concat_3/13
  Inport_278/1 -> Concat_3/14
  Inport_279/1 -> Concat_3/15
  Inport_280/1 -> Concat_3/16
  Inport_281/1 -> Concat_3/17
  Inport_282/1 -> Concat_3/18
  Inport_283/1 -> Concat_3/19
  Inport_284/1 -> Concat_3/20
  Inport_285/1 -> Concat_3/21
  Inport_286/1 -> Concat_3/22
  Inport_287/1 -> Concat_3/23
  Inport_288/1 -> Concat_3/24
  Inport_289/1 -> Concat_3/25
  Inport_290/1 -> Concat_3/26
  Inport_291/1 -> Concat_3/27
  Inport_292/1 -> Concat_3/28
  Inport_293/1 -> Concat_3/29
  Inport_294/1 -> Concat_3/30
  Inport_295/1 -> Concat_3/31
  Inport_296/1 -> Concat_3/32
  Inport_297/1 -> Concat_3/33
  Inport_298/1 -> Concat_3/34
  Inport_299/1 -> Concat_3/35
  Inport_300/1 -> Concat_3/36
  Inport_301/1 -> Concat_3/37
  Inport_302/1 -> Concat_3/38
  Inport_303/1 -> Concat_3/39
  Inport_304/1 -> Concat_3/40
  Inport_305/1 -> Concat_3/41
  Inport_306/1 -> Concat_3/42
  Inport_307/1 -> Concat_3/43
  Inport_308/1 -> Concat_3/44
  Inport_309/1 -> Concat_3/45
  Inport_310/1 -> Concat_3/46
  Inport_311/1 -> Concat_3/47
  Inport_312/1 -> Concat_3/48
  SigSpec_44/1 -> Outport_44/1
  RateTs_44/1 -> SigSpec_44/1
  Data_Conversion_47/1 -> RateTs_44/1
  Inport_313/1 -> Data_Conversion_47/1
  SigSpec_45/1 -> Outport_45/1
  RateTs_45/1 -> SigSpec_45/1
  Data_Conversion_48/1 -> RateTs_45/1
  Inport_314/1 -> Data_Conversion_48/1
  SigSpec_46/1 -> Outport_46/1
  RateTs_46/1 -> SigSpec_46/1
  Data_Conversion_49/1 -> RateTs_46/1
  Inport_315/1 -> Data_Conversion_49/1
  SigSpec_47/1 -> Outport_47/1
  RateTs_47/1 -> SigSpec_47/1
  Data_Conversion_50/1 -> RateTs_47/1
  Inport_316/1 -> Data_Conversion_50/1
  SigSpec_48/1 -> Outport_48/1
  RateTs_48/1 -> SigSpec_48/1
  Data_Conversion_51/1 -> RateTs_48/1
  Inport_317/1 -> Data_Conversion_51/1
  SigSpec_49/1 -> Outport_49/1
  RateTs_49/1 -> SigSpec_49/1
  Data_Conversion_52/1 -> RateTs_49/1
  Inport_318/1 -> Data_Conversion_52/1
  SigSpec_50/1 -> Outport_50/1
  RateTs_50/1 -> SigSpec_50/1
  Data_Conversion_53/1 -> RateTs_50/1
  Inport_319/1 -> Data_Conversion_53/1
  SigSpec_51/1 -> Outport_51/1
  RateTs_51/1 -> SigSpec_51/1
  Data_Conversion_54/1 -> RateTs_51/1
  Inport_320/1 -> Data_Conversion_54/1
  SigSpec_52/1 -> Outport_52/1
  RateTs_52/1 -> SigSpec_52/1
  Data_Conversion_55/1 -> RateTs_52/1
  Inport_321/1 -> Data_Conversion_55/1
  SigSpec_53/1 -> Outport_53/1
  RateTs_53/1 -> SigSpec_53/1
  Data_Conversion_56/1 -> RateTs_53/1
  Inport_322/1 -> Data_Conversion_56/1
  SigSpec_54/1 -> Outport_54/1
  RateTs_54/1 -> SigSpec_54/1
  Data_Conversion_57/1 -> RateTs_54/1
  Inport_323/1 -> Data_Conversion_57/1
  SigSpec_55/1 -> Outport_55/1
  RateTs_55/1 -> SigSpec_55/1
  Data_Conversion_58/1 -> RateTs_55/1
  Inport_324/1 -> Data_Conversion_58/1
  SigSpec_56/1 -> Outport_56/1
  RateTs_56/1 -> SigSpec_56/1
  Data_Conversion_59/1 -> RateTs_56/1
  Inport_325/1 -> Data_Conversion_59/1
  SigSpec_57/1 -> Outport_57/1
  RateTs_57/1 -> SigSpec_57/1
  Data_Conversion_60/1 -> RateTs_57/1
  Inport_326/1 -> Data_Conversion_60/1
  SigSpec_58/1 -> Outport_58/1
  RateTs_58/1 -> SigSpec_58/1
  Data_Conversion_61/1 -> RateTs_58/1
  Inport_327/1 -> Data_Conversion_61/1
  SigSpec_59/1 -> Outport_59/1
  RateTs_59/1 -> SigSpec_59/1
  Data_Conversion_62/1 -> RateTs_59/1
  Inport_328/1 -> Data_Conversion_62/1
  SigSpec_60/1 -> Outport_60/1
  RateTs_60/1 -> SigSpec_60/1
  Data_Conversion_63/1 -> RateTs_60/1
  Inport_329/1 -> Data_Conversion_63/1
  SigSpec_61/1 -> Outport_61/1
  RateTs_61/1 -> SigSpec_61/1
  Data_Conversion_64/1 -> RateTs_61/1
  Inport_330/1 -> Data_Conversion_64/1
  SigSpec_62/1 -> Outport_62/1
  RateTs_62/1 -> SigSpec_62/1
  Data_Conversion_65/1 -> RateTs_62/1
  Inport_331/1 -> Data_Conversion_65/1
  SigSpec_63/1 -> Outport_63/1
  RateTs_63/1 -> SigSpec_63/1
  Data_Conversion_66/1 -> RateTs_63/1
  Inport_332/1 -> Data_Conversion_66/1
  SigSpec_64/1 -> Outport_64/1
  RateTs_64/1 -> SigSpec_64/1
  Data_Conversion_67/1 -> RateTs_64/1
  Inport_333/1 -> Data_Conversion_67/1
  SigSpec_65/1 -> Outport_65/1
  RateTs_65/1 -> SigSpec_65/1
  Data_Conversion_68/1 -> RateTs_65/1
  Inport_334/1 -> Data_Conversion_68/1
  SigSpec_66/1 -> Outport_66/1
  RateTs_66/1 -> SigSpec_66/1
  Data_Conversion_69/1 -> RateTs_66/1
  Inport_335/1 -> Data_Conversion_69/1
  SigSpec_67/1 -> Outport_67/1
  RateTs_67/1 -> SigSpec_67/1
  Data_Conversion_70/1 -> RateTs_67/1
  Inport_336/1 -> Data_Conversion_70/1
  SigSpec_68/1 -> Outport_68/1
  RateTs_68/1 -> SigSpec_68/1
  Data_Conversion_71/1 -> RateTs_68/1
  Inport_337/1 -> Data_Conversion_71/1
  SigSpec_69/1 -> Outport_69/1
  RateTs_69/1 -> SigSpec_69/1
  Data_Conversion_72/1 -> RateTs_69/1
  Inport_338/1 -> Data_Conversion_72/1
  SigSpec_70/1 -> Outport_70/1
  RateTs_70/1 -> SigSpec_70/1
  Data_Conversion_73/1 -> RateTs_70/1
  Inport_339/1 -> Data_Conversion_73/1
  SigSpec_71/1 -> Outport_71/1
  RateTs_71/1 -> SigSpec_71/1
  Data_Conversion_74/1 -> RateTs_71/1
  Inport_340/1 -> Data_Conversion_74/1
  SigSpec_72/1 -> Outport_72/1
  RateTs_72/1 -> SigSpec_72/1
  Data_Conversion_75/1 -> RateTs_72/1
  Inport_341/1 -> Data_Conversion_75/1
  SigSpec_73/1 -> Outport_73/1
  RateTs_73/1 -> SigSpec_73/1
  Data_Conversion_76/1 -> RateTs_73/1
  Inport_342/1 -> Data_Conversion_76/1
  SigSpec_74/1 -> Outport_74/1
  RateTs_74/1 -> SigSpec_74/1
  Data_Conversion_77/1 -> RateTs_74/1
  Inport_343/1 -> Data_Conversion_77/1
  SigSpec_75/1 -> Outport_75/1
  RateTs_75/1 -> SigSpec_75/1
  Data_Conversion_78/1 -> RateTs_75/1
  Inport_344/1 -> Data_Conversion_78/1
  SigSpec_76/1 -> Outport_76/1
  RateTs_76/1 -> SigSpec_76/1
  Data_Conversion_79/1 -> RateTs_76/1
  Inport_345/1 -> Data_Conversion_79/1
  SigSpec_77/1 -> Outport_77/1
  RateTs_77/1 -> SigSpec_77/1
  Data_Conversion_80/1 -> RateTs_77/1
  Inport_346/1 -> Data_Conversion_80/1
  SigSpec_78/1 -> Outport_78/1
  RateTs_78/1 -> SigSpec_78/1
  Data_Conversion_81/1 -> RateTs_78/1
  Data_Conversion_82/1 -> Data_Conversion_81/1
  Concat_4/1 -> Data_Conversion_82/1
  Inport_347/1 -> Concat_4/1
  Inport_348/1 -> Concat_4/2
  Inport_349/1 -> Concat_4/3
  Inport_350/1 -> Concat_4/4
  Inport_351/1 -> Concat_4/5
  Inport_352/1 -> Concat_4/6
  Inport_353/1 -> Concat_4/7
  Inport_354/1 -> Concat_4/8
  Inport_355/1 -> Concat_4/9
  Inport_356/1 -> Concat_4/10
  Inport_357/1 -> Concat_4/11
  Inport_358/1 -> Concat_4/12
  Inport_359/1 -> Concat_4/13
  Inport_360/1 -> Concat_4/14
  Inport_361/1 -> Concat_4/15
  Inport_362/1 -> Concat_4/16
  Inport_363/1 -> Concat_4/17
  Inport_364/1 -> Concat_4/18
  Inport_365/1 -> Concat_4/19
  Inport_366/1 -> Concat_4/20
  Inport_367/1 -> Concat_4/21
  Inport_368/1 -> Concat_4/22
  Inport_369/1 -> Concat_4/23
  Inport_370/1 -> Concat_4/24
  Inport_371/1 -> Concat_4/25
  Inport_372/1 -> Concat_4/26
  Inport_373/1 -> Concat_4/27
  Inport_374/1 -> Concat_4/28
  Inport_375/1 -> Concat_4/29
  Inport_376/1 -> Concat_4/30
  Inport_377/1 -> Concat_4/31
  Inport_378/1 -> Concat_4/32
  Inport_379/1 -> Concat_4/33
  Inport_380/1 -> Concat_4/34
  Inport_381/1 -> Concat_4/35
  Inport_382/1 -> Concat_4/36
  Inport_383/1 -> Concat_4/37
  Inport_384/1 -> Concat_4/38
  Inport_385/1 -> Concat_4/39
  Inport_386/1 -> Concat_4/40
  Inport_387/1 -> Concat_4/41
  Inport_388/1 -> Concat_4/42
  Inport_389/1 -> Concat_4/43
  Inport_390/1 -> Concat_4/44
  Inport_391/1 -> Concat_4/45
  Inport_392/1 -> Concat_4/46
  Inport_393/1 -> Concat_4/47
  Inport_394/1 -> Concat_4/48
  SigSpec_79/1 -> Outport_79/1
  RateTs_79/1 -> SigSpec_79/1
  Data_Conversion_83/1 -> RateTs_79/1
  Inport_395/1 -> Data_Conversion_83/1
  SigSpec_80/1 -> Outport_80/1
  RateTs_80/1 -> SigSpec_80/1
  Data_Conversion_84/1 -> RateTs_80/1
  Inport_396/1 -> Data_Conversion_84/1
  SigSpec_81/1 -> Outport_81/1
  RateTs_81/1 -> SigSpec_81/1
  Data_Conversion_85/1 -> RateTs_81/1
  Inport_397/1 -> Data_Conversion_85/1
  SigSpec_82/1 -> Outport_82/1
  RateTs_82/1 -> SigSpec_82/1
  Data_Conversion_86/1 -> RateTs_82/1
  Inport_398/1 -> Data_Conversion_86/1
  SigSpec_83/1 -> Outport_83/1
  RateTs_83/1 -> SigSpec_83/1
  Data_Conversion_87/1 -> RateTs_83/1
  Inport_399/1 -> Data_Conversion_87/1
  SigSpec_84/1 -> Outport_84/1
  RateTs_84/1 -> SigSpec_84/1
  Data_Conversion_88/1 -> RateTs_84/1
  Inport_400/1 -> Data_Conversion_88/1
  SigSpec_85/1 -> Outport_85/1
  RateTs_85/1 -> SigSpec_85/1
  Data_Conversion_89/1 -> RateTs_85/1
  Inport_401/1 -> Data_Conversion_89/1
  SigSpec_86/1 -> Outport_86/1
  RateTs_86/1 -> SigSpec_86/1
  Data_Conversion_90/1 -> RateTs_86/1
  Inport_402/1 -> Data_Conversion_90/1
  SigSpec_87/1 -> Outport_87/1
  RateTs_87/1 -> SigSpec_87/1
  Data_Conversion_91/1 -> RateTs_87/1
  Inport_403/1 -> Data_Conversion_91/1
  SigSpec_88/1 -> Outport_88/1
  RateTs_88/1 -> SigSpec_88/1
  Data_Conversion_92/1 -> RateTs_88/1
  Inport_404/1 -> Data_Conversion_92/1
  SigSpec_89/1 -> Outport_89/1
  RateTs_89/1 -> SigSpec_89/1
  Data_Conversion_93/1 -> RateTs_89/1
  Inport_405/1 -> Data_Conversion_93/1
  SigSpec_90/1 -> Outport_90/1
  RateTs_90/1 -> SigSpec_90/1
  Data_Conversion_94/1 -> RateTs_90/1
  Inport_406/1 -> Data_Conversion_94/1
  SigSpec_91/1 -> Outport_91/1
  RateTs_91/1 -> SigSpec_91/1
  Data_Conversion_95/1 -> RateTs_91/1
  Inport_407/1 -> Data_Conversion_95/1
  SigSpec_92/1 -> Outport_92/1
  RateTs_92/1 -> SigSpec_92/1
  Data_Conversion_96/1 -> RateTs_92/1
  Inport_408/1 -> Data_Conversion_96/1
  SigSpec_93/1 -> Outport_93/1
  RateTs_93/1 -> SigSpec_93/1
  Data_Conversion_97/1 -> RateTs_93/1
  Inport_409/1 -> Data_Conversion_97/1
  SigSpec_94/1 -> Outport_94/1
  RateTs_94/1 -> SigSpec_94/1
  Data_Conversion_98/1 -> RateTs_94/1
  Inport_410/1 -> Data_Conversion_98/1
  SigSpec_95/1 -> Outport_95/1
  RateTs_95/1 -> SigSpec_95/1
  Data_Conversion_99/1 -> RateTs_95/1
  Inport_411/1 -> Data_Conversion_99/1
  SigSpec_96/1 -> Outport_96/1
  RateTs_96/1 -> SigSpec_96/1
  Data_Conversion_100/1 -> RateTs_96/1
  Inport_412/1 -> Data_Conversion_100/1
  SigSpec_97/1 -> Outport_97/1
  RateTs_97/1 -> SigSpec_97/1
  Data_Conversion_101/1 -> RateTs_97/1
  Inport_413/1 -> Data_Conversion_101/1
